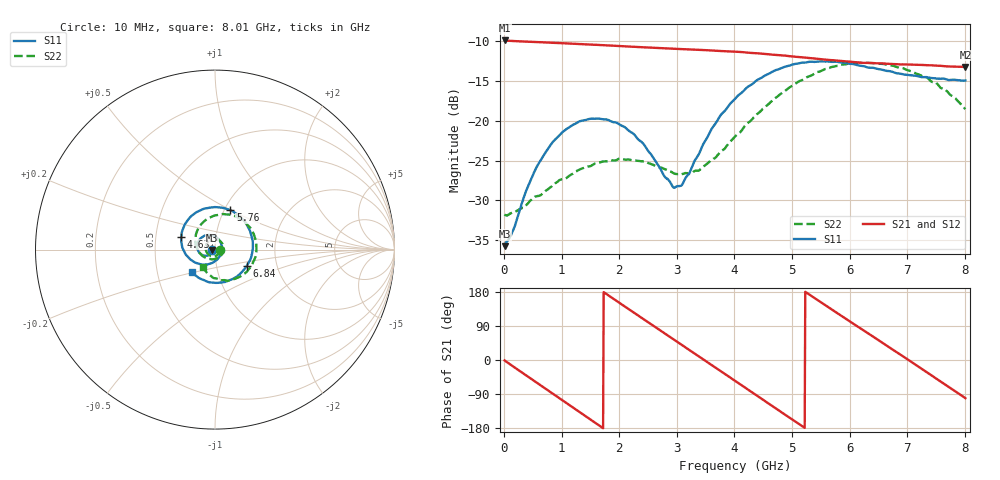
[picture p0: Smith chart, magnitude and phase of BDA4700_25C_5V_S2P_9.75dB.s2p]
!Agilent Technologies,E5071B,MY42404982,A.09.10
!Date: Mon Oct 20 13:30:55 2025
!Data & Calibration Information:
!Freq	S11:SOLT2(ON)	S21:SOLT2(ON)	S12:SOLT2(ON)	S22:SOLT2(ON)
# Hz S RI R 50
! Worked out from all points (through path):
!   801 points, 10 MHz to 8.01 GHz, reference 50 ohm
!   highest |S21| = -9.87 dB at 10 MHz (marker M1); lowest = -13.2 dB at 8.01 GHz (marker M2)
!   group delay of S21, straight-line fit = 284 ps
!   lowest |S11| = -35.8 dB at 10 MHz (marker M3), VSWR 1.03, Z = 48.4 - j0.128 ohm
!   |S11| at or under -10 dB: start of sweep to end of sweep
!   |S22| runs from -31.9 to -12.7 dB; largest |S21 - S12| = 0.0025
!   S11 on the Smith chart (normalised r, x): 10 MHz: 0.97, -0.00; 4.63 GHz: 0.68, +0.10; 5.76 GHz: 1.07, +0.50; 6.84 GHz: 1.41, -0.26; 8.01 GHz: 0.75, -0.19
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1e7  -0.0162 -0.00132  0.3209 -0.00701  0.3208 -0.00714  0.0258 -0.00134
3.3e8  -0.0236 -0.0215  0.2585 -0.1822  0.2583 -0.1825  0.022 -0.018
7.1e8  -0.052 -0.0345  0.0809 -0.3012  0.0807 -0.3014  0.000791 -0.036
1.02e9  -0.0823 -0.0224  -0.0917 -0.2943  -0.0918 -0.2945  -0.0265 -0.0339
1.35e9  -0.0997 0.0118  -0.2384 -0.189  -0.2386 -0.1892  -0.0494 -0.00794
1.93e9  -0.0623 0.0754  -0.2761 0.1095  -0.2761 0.1095  -0.0268 0.0496
2.32e9  -0.00891 0.0766  -0.1384 0.2571  -0.1384 0.2572  0.0173 0.0535
2.68e9  0.0302 0.0427  0.0428 0.2847  0.0427 0.2846  0.0457 0.0228
2.93e9  0.0382 0.00486  0.16 0.2359  0.1599 0.2356  0.0468 -0.0056
3.07e9  0.0348 -0.0178  0.2126 0.1877  0.2116 0.1885  0.0408 -0.0218
3.53e9  -0.0208 -0.0761  0.2771 -0.0268  0.2773 -0.0272  -0.00664 -0.0535
4.01e9  -0.1205 -0.0663  0.157 -0.223  0.1573 -0.2227  -0.0723 -0.0331
4.32e9  -0.1714 -0.00995  0.0156 -0.2669  0.0154 -0.2677  -0.1028 0.0125
4.63e9  -0.1872 0.0727  -0.1258 -0.2298  -0.1255 -0.2301  -0.1074 0.0764
5e9  -0.1448 0.1733  -0.2336 -0.1015  -0.2342 -0.1016  -0.0659 0.1528
5.35e9  -0.0505 0.2302  -0.2422 0.0528  -0.2425 0.052  0.0185 0.1931
5.76e9  0.0858 0.2198  -0.1421 0.1933  -0.142 0.1936  0.1362 0.1747
6.19e9  0.1879 0.119  0.0266 0.231  0.0285 0.2312  0.2203 0.0733
6.68e9  0.202 -0.0408  0.189 0.1288  0.1893 0.1287  0.2126 -0.0703
6.84e9  0.1784 -0.0886  0.2157 0.0714  0.216 0.0702  0.1873 -0.1099
7.33e9  0.0555 -0.1805  0.1916 -0.1165  0.1916 -0.117  0.0731 -0.1733
8.01e9  -0.1308 -0.1233  -0.041 -0.2146  -0.0407 -0.2148  -0.0677 -0.0974
